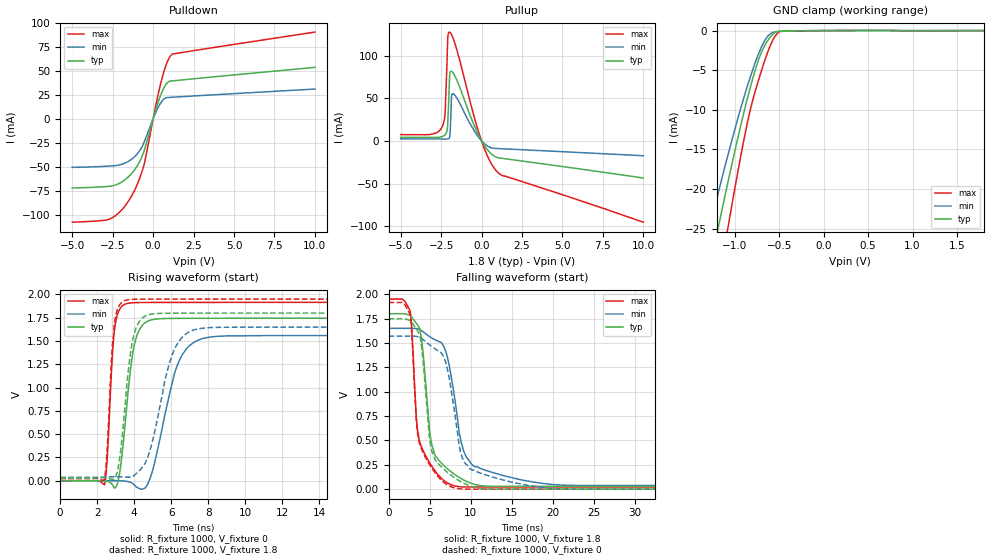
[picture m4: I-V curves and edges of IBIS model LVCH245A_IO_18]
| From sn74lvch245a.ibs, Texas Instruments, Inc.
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[Model]   LVCH245A_IO_18
Model_type  I/O
Vinl=0.5775
Vinh=1.2675
Enable   Active-Low
Vref =   0
Rref =   1000
Cref =   30p
Vmeas =   0.9
| variable   typ   min   max
C_comp   4.48pF   4.24pF   5.07pF
| C_pullup   6.02pF   5.29pF   6.45pF
| C_pulldown   5.77pF   3.89pF   7.20pF
| C_tri-state   4.48pF   4.24pF   5.07pF
[Temperature Range]   40   100   -40
| Ambient temperature   25   85   -40
[Voltage range]   1.8   1.65   1.95
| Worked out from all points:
|   slope of the pulldown table from 0 to 0.27 V, typ, clamps not added: 17.6 ohm
|   slope of the pullup table from 0 to 0.27 V, typ, clamps not added: 33.3 ohm
|   GND clamp passes 1 mA (typ) near -0.61 V on its own axis
|   rising waveform, R_fixture 1000, V_fixture 0: 20-80 % time 563ps typ, 1.11ns min, 309ps max; typ from 0 V to 1.75 V
|   falling waveform, R_fixture 1000, V_fixture 1.8: 20-80 % time 1.38ns typ, 2.06ns min, 1.26ns max; typ from 1.8 V to 0.029 V
|   rising waveform, R_fixture 1000, V_fixture 1.8: 20-80 % time 555ps typ, 1.11ns min, 303ps max; typ from 0.029 V to 1.8 V
|   falling waveform, R_fixture 1000, V_fixture 0: 20-80 % time 1.35ns typ, 1.92ns min, 1.29ns max; typ from 1.75 V to 0 V
[GND Clamp]
| LVCH245A_IO_18
|   Voltage   I(typ)   I(min)   I(max)
-5V       -263.5mA   -221.8mA   -330.8mA
-1.27V    -29.51mA   -24.36mA   -37.97mA
-1.19V    -25.16mA   -20.72mA   -32.49mA
-1.15V    -23.02mA   -18.94mA   -29.79mA
-1.08V    -19.35mA   -15.89mA   -25.16mA
-1.045V   -17.56mA   -14.4mA    -22.89mA
-855mV    -8.478mA   -6.92mA    -11.53mA
-745mV    -4.131mA   -3.311mA   -6.747mA
-630mV    -1.28mA    -735.5uA   -2.76mA
-570mV    -464.7uA   -244.6uA   -1.178mA
-510mV    -87.77uA   -112.1uA   -243.6uA
1.8V      16.54pA    66.02nA    -2.716nA
[Pulldown]
| LVCH245A_IO_18
|   Voltage   I(typ)   I(min)   I(max)
-5V       -72.08mA   -50.56mA   -107.8mA
-2.685V   -70.3mA    -49.18mA   -104.4mA
-2.025V   -66.64mA   -47.78mA   -96.4mA
-1.395V   -58.12mA   -42.82mA   -82.22mA
-1V       -49.45mA   -36.89mA   -68.93mA
-600mV    -35.53mA   -26.02mA   -50.16mA
-485mV    -29.38mA   -21.15mA   -42.12mA
130mV     7.726mA    5.46mA     11.19mA
480mV     25.3mA     16.98mA    37.67mA
835mV     36.82mA    22.16mA    57.63mA
1.15V     39.54mA    22.49mA    67.01mA
10V       53.67mA    31.09mA    90.48mA
[Pullup]
| LVCH245A_IO_18
|   Voltage   I(typ)   I(min)   I(max)
-5V       4.242mA    2.356mA    7.385mA
-2.43V    5.003mA    2.203mA    16.63mA
-2.25V    7.24mA     2.191mA    33.49mA
-2.11V    14.75mA    2.227mA    107.3mA
-2.075V   26.71mA    2.329mA    123.4mA
-1.975V   75.44mA    3.957mA    127.6mA
-1.925V   81.07mA    16.17mA    126.8mA
-1.855V   81.55mA    52.16mA    124.6mA
-1.755V   79.65mA    55.16mA    120.2mA
-55mV     1.925mA    1.19mA     3.099mA
995mV     -19.66mA   -8.969mA   -36.76mA
10V       -43.52mA   -17.42mA   -95.35mA
[Ramp]
| LVCH245A_IO_18
| variable   typ   min   max
dV/dt_r   1.09/5.97E-10   0.99/1.21E-09   1.18/3.27E-10
dV/dt_f   1.06/1.44E-09   0.97/2.31E-09   1.16/1.27E-09
R_load = 1000
[Rising Waveform]
| LVCH245A_IO_18
R_fixture =   1000
C_fixture =   0
L_fixture =   0
V_fixture =   0
V_fixture_min = 0
V_fixture_max = 0
|   Time   V(typ)   V(min)   V(max)
0s        200pV      5.177nV    30.06nV
2.4ns     -1.025mV   -694.3uV   -43.92mV
2.945ns   -78.15mV   894.9uV    1.627V
3.255ns   133mV      -69.74uV   1.852V
3.665ns   942mV      -9.525mV   1.905V
4.025ns   1.471V     -47.22mV   1.911V
4.535ns   1.686V     -83.86mV   1.913V
6.405ns   1.743V     1.274V     1.914V
7.98ns    1.744V     1.539V     1.914V
50ns      1.745V     1.559V     1.915V
[Falling Waveform]
| LVCH245A_IO_18
R_fixture =   1000
C_fixture =   0
L_fixture =   0
V_fixture =   1.8
V_fixture_min = 1.65
V_fixture_max = 1.95
|   Time   V(typ)   V(min)   V(max)
0s        1.8V       1.65V      1.95V
2.64ns    1.781V     1.651V     1.824V
3.385ns   1.701V     1.647V     743.7mV
3.8ns     1.646V     1.637V     484.1mV
5.26ns    460.7mV    1.551V     236.7mV
6.615ns   252.5mV    1.481V     97.88mV
7.515ns   185.1mV    1.215V     49.12mV
9.16ns    93.99mV    391.5mV    22.1mV
11.58ns   32.37mV    199.5mV    22.11mV
50ns      28.98mV    37.19mV    21.86mV
[Rising Waveform]
| LVCH245A_IO_18
R_fixture =   1000
C_fixture =   0
L_fixture =   0
V_fixture =   1.8
V_fixture_min = 1.65
V_fixture_max = 1.95
|   Time   V(typ)   V(min)   V(max)
0s        28.92mV    37.03mV    21.84mV
2.4ns     32.3mV     40.53mV    19.68mV
2.92ns    17.44mV    42.65mV    1.668V
3.24ns    274.3mV    42.01mV    1.894V
3.64ns    1.095V     38.91mV    1.942V
3.96ns    1.544V     51.03mV    1.947V
4.44ns    1.746V     144.2mV    1.949V
6.125ns   1.798V     1.385V     1.95V
7.51ns    1.799V     1.632V     1.95V
50ns      1.8V       1.65V      1.95V
[Falling Waveform]
| LVCH245A_IO_18
R_fixture =   1000
C_fixture =   0
L_fixture =   0
V_fixture =   0
V_fixture_min = 0
V_fixture_max = 0
|   Time   V(typ)   V(min)   V(max)
0s        1.748V     1.57V      1.915V
2.64ns    1.728V     1.571V     1.785V
3.38ns    1.644V     1.568V     712mV
3.795ns   1.581V     1.557V     462.4mV
5.215ns   410.5mV    1.466V     223.3mV
6.64ns    212.5mV    1.369V     76.26mV
7.545ns   147.4mV    1.064V     27.09mV
9.125ns   62.46mV    293.2mV    489.6uV
12.65ns   -356.9uV   124.3mV    333.4uV
50ns      57.64uV    65.62uV    21.25uV
